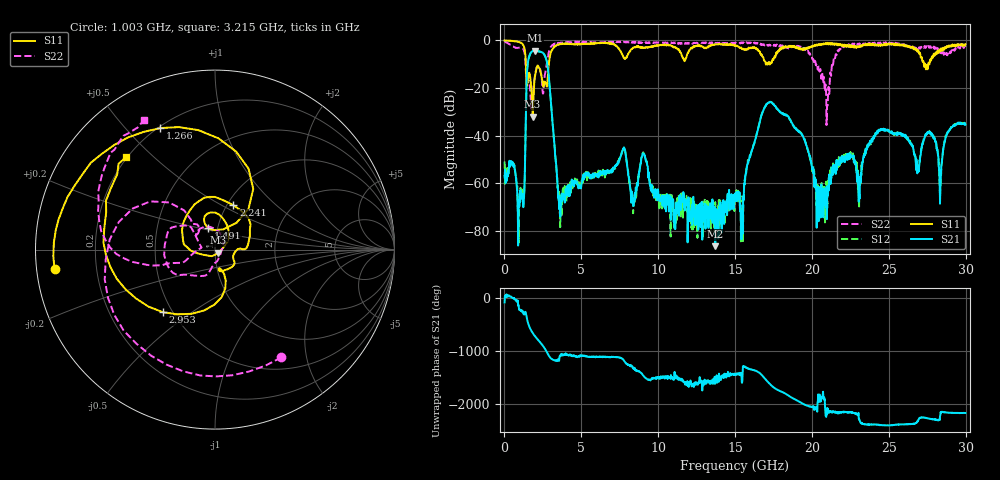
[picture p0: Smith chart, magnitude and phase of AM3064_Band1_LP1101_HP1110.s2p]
# Hz S DB R 50.0
!freq dBS11 angS11 dBS21 angS21 dBS12 angS12 dBS22 angS22
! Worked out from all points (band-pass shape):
!   1600 points, 10 MHz to 29.98 GHz, reference 50 ohm
!   highest |S21| = -4.27 dB at 1.978 GHz (marker M1); lowest = -86.4 dB at 13.71 GHz (marker M2)
!   |S21| within 3 dB of the highest: 1.587 GHz to 2.684 GHz (1.096 GHz wide, 51.3 % of centre)
!   lowest |S11| = -32.0 dB at 1.828 GHz (marker M3), VSWR 1.05, Z = 51.9 - j1.74 ohm
!   |S11| at or under -10 dB: 1.393 GHz to 2.883 GHz (1.49 GHz wide, 69.7 % of centre); 27.2807 GHz to 27.34913 GHz (68.43 MHz wide, 0.251 % of centre); 27.37 GHz to 27.57 GHz (204.7 MHz wide, 0.745 % of centre)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
!   |S22| runs from -35.5 to -0.4 dB; largest |S21 - S12| = 0.0092
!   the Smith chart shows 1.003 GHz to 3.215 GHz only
!   S11 on the Smith chart (normalised r, x): 1.003 GHz: 0.05, -0.06; 1.266 GHz: 0.21, +0.63; 1.491 GHz: 0.90, +0.22; 2.241 GHz: 1.07, +0.57; 2.953 GHz: 0.44, -0.39; 3.215 GHz: 0.19, +0.41
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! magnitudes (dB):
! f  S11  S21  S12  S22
! 10 MHz  -0.1  -56.9  -50.8  -0.4
! 1.003 GHz  -0.9  -64.0  -64.6  -3.0
! 1.266 GHz  -2.6  -65.7  -65.8  -4.3
! 1.491 GHz  -18.0  -11.3  -11.2  -17.2
! 1.828 GHz  -32.0  -4.5  -4.5  -23.5
! 1.978 GHz  -15.1  -4.3  -4.3  -15.6
! 2.241 GHz  -11.5  -4.7  -4.6  -11.1
! 2.953 GHz  -6.9  -20.4  -20.4  -3.6
! 3.215 GHz  -2.9  -41.0  -41.3  -1.7
! 3.609 GHz  -1.7  -70.4  -73.0  -1.2
! 5.015 GHz  -1.6  -60.3  -58.5  -0.6
! 7.751 GHz  -7.2  -45.6  -44.8  -0.6
! 8.351 GHz  -3.1  -66.4  -65.6  -0.7
! 10 GHz  -2.1  -63.5  -66.5  -0.9
! 13.71 GHz  -1.7  -86.4  -67.9  -1.3
! 15 GHz  -2.3  -65.1  -67.5  -1.3
! 17.2 GHz  -9.1  -26.2  -26.1  -1.9
! 19.99 GHz  -2.9  -52.8  -52.7  -6.8
! 20.76 GHz  -1.3  -62.0  -72.7  -15.8
! 25 GHz  -1.4  -38.0  -37.7  -1.3
! 28.35 GHz  -4.7  -61.7  -62.9  -5.4
! 29.98 GHz  -1.7  -35.4  -35.4  -2.9
